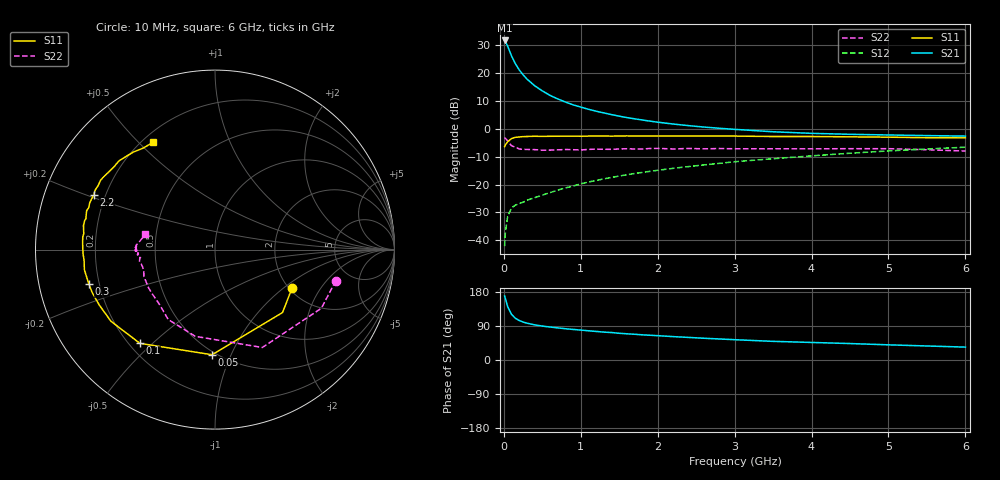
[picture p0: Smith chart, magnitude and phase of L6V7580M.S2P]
!  INFINEON TECHNOLOGIES Small Signal Semiconductors
! BFR380L3 , Si-NPN RF-Transistor in TSLP-3-1
!  Vce=0.75 V,  Ic=80 mA
! Common Emitter S-Parameters:  07. March 2005
#  GHz  S  MA  R  50
! f  S11  S21  S12  S22
! GHz  Mag  Ang  Mag  Ang  Mag  Ang  Mag  Ang
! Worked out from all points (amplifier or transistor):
!   36 points, 10 MHz to 6 GHz, reference 50 ohm
!   highest |S21| = 31.8 dB at 10 MHz (marker M1)
!   |S21| within 3 dB of that: start of sweep to 62.91 MHz
!   unconditionally stable (mu >= 1): 647.3 MHz to end of sweep
!   at 250 MHz: K = 0.63, MSG = 22.9 dB, |S12| = -26.4 dB
!   at 1.4 GHz: K = 1.15, MAG = 9.0 dB, |S12| = -17.5 dB
!   at 6 GHz: K = 1.06, MAG = 0.6 dB, |S12| = -6.6 dB
!   S11 on the Smith chart (normalised r, x): 10 MHz: 2.06, -1.16; 50 MHz: 0.48, -0.85; 100 MHz: 0.24, -0.46; 300 MHz: 0.16, -0.13; 2.2 GHz: 0.16, +0.21; 6 GHz: 0.24, +0.55
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0.01  0.4803 -26.8  38.73 169.0  0.0078 56.6  0.6954 -14.4
0.02  0.5143 -43.0  37.27 162.3  0.0138 61.9  0.6766 -28.9
0.05  0.5861 -91.6  30.38 140.5  0.0267 52.3  0.6058 -64.2
0.1  0.6693 -128.7  20.43 120.4  0.0381 41.2  0.4956 -102.8
0.15  0.7038 -145.4  14.78 110.1  0.0426 37.8  0.4686 -123.8
0.2  0.7149 -154.3  11.47 104.3  0.0454 39.4  0.4349 -135.2
0.25  0.725 -160.8  9.375 100.2  0.0481 39.4  0.4278 -145.4
0.3  0.7286 -164.8  7.855 97.2  0.0521 42.0  0.4271 -150.1
0.4  0.7363 -171.2  5.96 92.7  0.0578 45.6  0.4234 -159.3
0.5  0.7319 -175.4  4.804 89.6  0.0644 49.4  0.4133 -163.6
0.6  0.7354 -178.1  3.992 87.0  0.0714 52.3  0.4146 -166.5
0.7  0.7368 179.5  3.451 84.7  0.0792 54.8  0.4193 -169.3
0.8  0.7387 176.7  3.035 82.5  0.0868 56.2  0.4255 -171.2
0.9  0.7401 174.5  2.698 80.7  0.0937 58.0  0.422 -173.3
1.1  0.741 171.2  2.245 77.1  0.1109 60.2  0.4272 -174.3
1.3  0.7439 167.3  1.93 73.6  0.1266 61.1  0.4294 -177.7
1.6  0.7473 163.1  1.594 69.1  0.1496 61.9  0.4393 -179.2
2.2  0.7415 155.7  1.222 61.7  0.1952 62.1  0.4352 -179.7
3.5  0.7278 140.9  0.886 49.2  0.2903 58.9  0.4389 178.0
4.5  0.7186 134.1  0.798 43.4  0.3646 55.6  0.4402 177.1
5.5  0.6927 125.3  0.756 37.0  0.4348 50.2  0.4214 173.6
6  0.69 120.1  0.741 34.0  0.4679 47.6  0.3985 167.8
